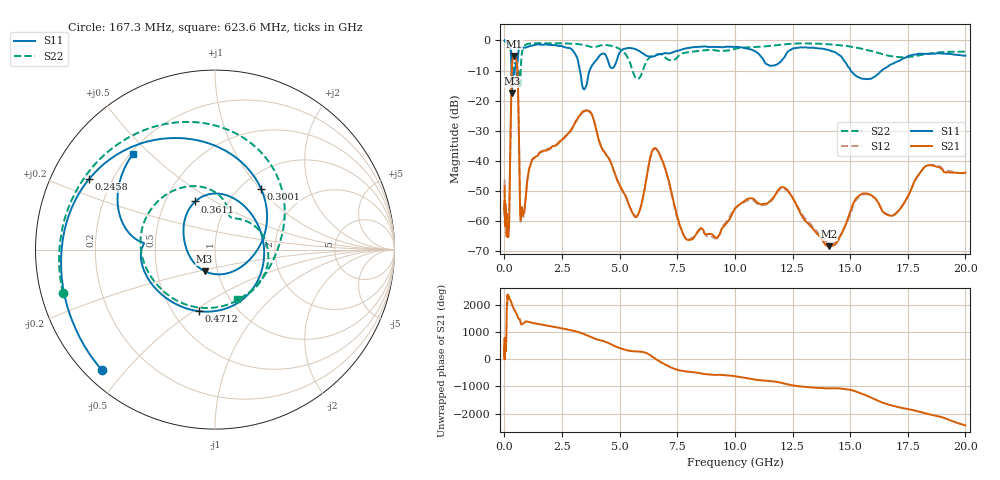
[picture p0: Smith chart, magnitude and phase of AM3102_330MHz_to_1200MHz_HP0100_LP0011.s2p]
! Date/Time: Tue, Sep 11, 2018 5:12 PM
! Network Analyzer: Agilent Technologies E8362B Rev: A.07.50.63
! Sweep from 0.010 to 20.000 GHz, 1601 Points, Sweep Type: LOG
! Power Supply: 4.949 V, 0.001 A
# Hz S DB R 50
!freq MagS11 AngS11 MagS21 AngS21 MagS12 AngS12 MagS22 AngS22
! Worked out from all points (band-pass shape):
!   1601 points, 10 MHz to 20 GHz, reference 50 ohm
!   highest |S21| = -5.17 dB at 416.5 MHz (marker M1); lowest = -68.3 dB at 14.07 GHz (marker M2)
!   |S21| within 3 dB of the highest: 332.8 MHz to 552 MHz (219.2 MHz wide, 49.5 % of centre)
!   lowest |S11| = -17.5 dB at 330 MHz (marker M3), VSWR 1.31, Z = 43.3 - j10.6 ohm
!   |S11| at or under -10 dB: 307.9 MHz to 446.7 MHz (138.9 MHz wide, 36.8 % of centre); 3.281 GHz to 3.695 GHz (414.1 MHz wide, 11.9 % of centre); 15.03 GHz to 16.37 GHz (1.346 GHz wide, 8.58 % of centre)
!   |S22| runs from -15.9 to -0.2 dB; largest |S21 - S12| = 0.013
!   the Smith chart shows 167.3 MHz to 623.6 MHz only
!   S11 on the Smith chart (normalised r, x): 167.3 MHz: 0.05, -0.43; 245.8 MHz: 0.12, +0.26; 300.1 MHz: 1.24, +1.01; 361.1 MHz: 0.70, +0.41; 471.2 MHz: 0.67, -0.53; 623.6 MHz: 0.21, +0.44
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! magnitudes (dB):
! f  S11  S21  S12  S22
! 10 MHz  0.0  -48.4  -46.1  -0.2
! 35.55 MHz  0.0  -57.7  -59.3  -0.4
! 126.4 MHz  -0.4  -64.6  -62.1  -0.9
! 167.3 MHz  -0.7  -65.3  -62.8  -1.1
! 245.8 MHz  -1.9  -41.3  -41.4  -2.0
! 300.1 MHz  -7.5  -16.7  -16.7  -4.5
! 330 MHz  -17.5  -8.6  -8.6  -8.6
! 361.1 MHz  -10.8  -6.1  -6.2  -10.3
! 416.5 MHz  -11.3  -5.2  -5.2  -8.3
! 447.2 MHz  -10.0  -5.3  -5.4  -7.5
! 471.2 MHz  -9.0  -5.5  -5.6  -7.5
! 561.8 MHz  -7.6  -9.3  -9.4  -14.0
! 623.6 MHz  -3.1  -28.1  -28.1  -10.4
! 705.6 MHz  -2.3  -59.6  -60.2  -10.9
! 1.59 GHz  -1.4  -36.9  -37.0  -0.9
! 3.651 GHz  -11.1  -23.4  -23.2  -1.9
! 5.652 GHz  -2.8  -58.4  -58.3  -11.9
! 6.58 GHz  -4.9  -35.9  -36.1  -4.8
! 7.958 GHz  -2.5  -66.2  -66.1  -3.9
! 12.09 GHz  -6.1  -48.7  -49.2  -1.4
! 14.07 GHz  -3.2  -68.3  -67.6  -1.3
! 20 GHz  -5.0  -43.9  -44.2  -3.7
